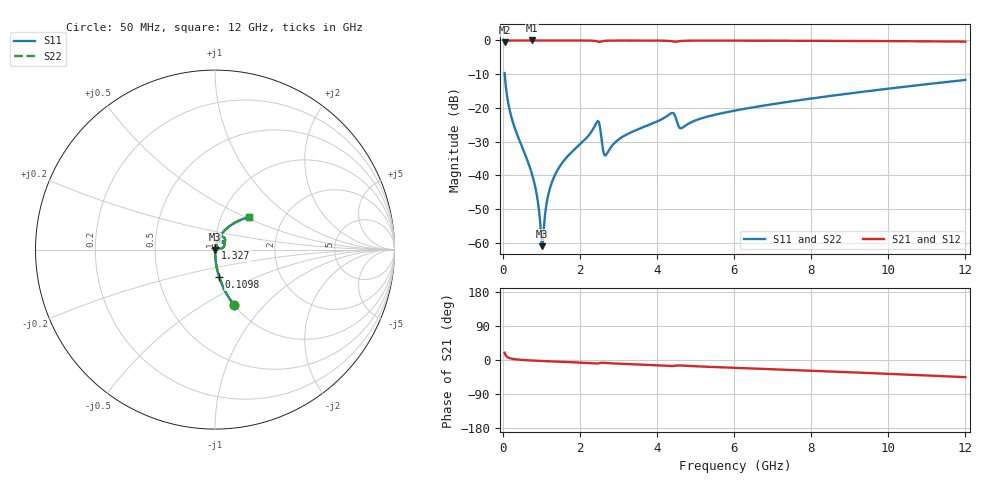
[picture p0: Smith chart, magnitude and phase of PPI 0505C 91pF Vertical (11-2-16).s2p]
# GHz S MA R 50
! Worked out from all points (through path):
!   1601 points, 50 MHz to 12 GHz, reference 50 ohm
!   highest |S21| = -0.01 dB at 752.1 MHz (marker M1); lowest = -0.5 dB at 50 MHz (marker M2)
!   group delay of S21, straight-line fit = 10.8 ps
!   lowest |S11| = -61.0 dB at 1.021 GHz (marker M3), VSWR 1.00, Z = 50.1 - j0.0149 ohm
!   |S11| at or under -10 dB: 52.24 MHz to end of sweep
!   |S22| runs from -61.0 to -9.7 dB; largest |S21 - S12| = 0
!   S11 on the Smith chart (normalised r, x): 50 MHz: 1.00, -0.70; 109.8 MHz: 1.00, -0.31; 1.327 GHz: 1.00, +0.02; 12 GHz: 1.35, +0.52
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0.05  0.3285 -70.9  0.9442 19.0  0.9442 19.0  0.3285 -70.9
0.10975  0.1551 -81.2  0.9875 8.6  0.9875 8.6  0.1551 -81.2
0.2740625  0.05901 -86.8  0.9977 2.7  0.9977 2.7  0.05901 -86.8
0.7520625  0.01082 -87.2  0.9991 -1.3  0.9991 -1.3  0.01082 -87.2
0.8790313  0.005365 -83.1  0.9991 -2.0  0.9991 -2.0  0.005365 -83.1
0.9835938  0.001651 -60.6  0.9991 -2.5  0.9991 -2.5  0.001651 -60.6
1.020938  0.0008933 -9.6  0.999 -2.6  0.999 -2.6  0.0008933 -9.6
1.058281  0.001457 48.9  0.999 -2.8  0.999 -2.8  0.001457 48.9
1.177781  0.005012 75.7  0.999 -3.3  0.999 -3.3  0.005012 75.7
1.327156  0.009351 79.8  0.9988 -4.0  0.9988 -4.0  0.009351 79.8
2.044156  0.03032 79.2  0.9974 -7.0  0.9974 -7.0  0.03032 79.2
2.462406  0.06359 45.4  0.9618 -9.3  0.9618 -9.3  0.06359 45.4
2.61925  0.02158 25.4  0.9816 -7.4  0.9816 -7.4  0.02158 25.4
2.679  0.02009 49.7  0.9889 -7.9  0.9889 -7.9  0.02009 49.7
3.09725  0.03694 75.4  0.9962 -10.1  0.9962 -10.1  0.03694 75.4
4.038312  0.06417 72.4  0.9938 -14.1  0.9938 -14.1  0.06417 72.4
4.404281  0.0843 54.3  0.968 -15.9  0.968 -15.9  0.0843 54.3
4.643281  0.05023 57.5  0.9832 -14.7  0.9832 -14.7  0.05023 57.5
6.025  0.09131 67.7  0.9929 -20.7  0.9929 -20.7  0.09131 67.7
8.019156  0.1382 60.5  0.9872 -28.4  0.9872 -28.4  0.1382 60.5
10.01331  0.1932 52.5  0.9774 -36.5  0.9774 -36.5  0.1932 52.5
12  0.2597 43.9  0.9613 -45.3  0.9613 -45.3  0.2597 43.9
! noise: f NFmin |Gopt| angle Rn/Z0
0.05  0.00037  0.858  0.3638  0.0005573
1.372  0.003835  0.6633  3.495  0.002179
2.701  0.01576  0.8233  6.952  0.01865
4.031  0.0126  0.6942  10.13  0.007974
5.36  0.01298  0.6227  13.27  0.006344
6.682  0.01345  0.5639  16.07  0.005451
8.012  0.01523  0.5457  18.92  0.005821
9.341  0.01728  0.5377  21.72  0.006405
10.67  0.01952  0.5356  24.46  0.007127
12  0.02196  0.538  27.15  0.007996
